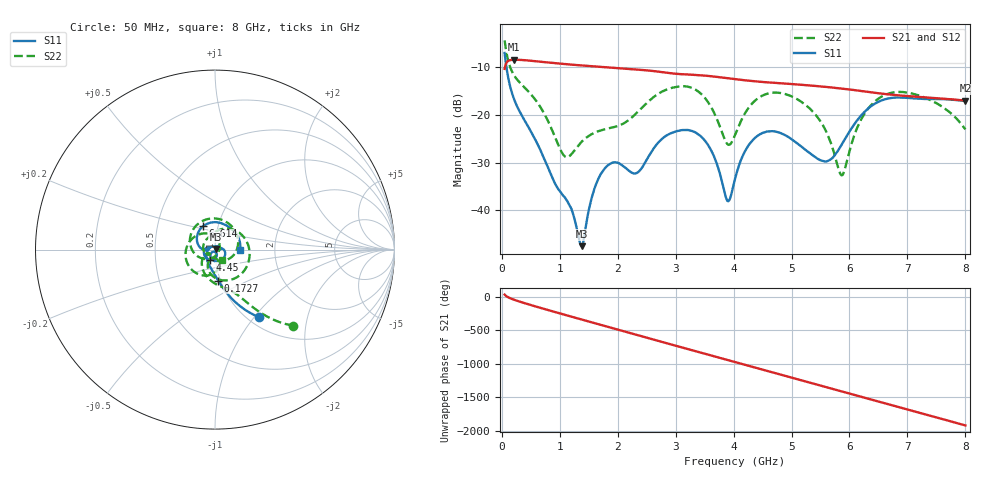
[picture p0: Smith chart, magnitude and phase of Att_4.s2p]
#  HZ  S  DB  R  50.00
! Rohde & Schwarz Vector Network Analyzer
! Rohde-Schwarz,ZNB40-4Port,1311601084101679,3.45
! Created: UTC 4/25/2025, 9:29:52 AM
! freq[Hz]  db:S11  ang:S11  db:S21  ang:S21  db:S12  ang:S12  db:S22  ang:S22
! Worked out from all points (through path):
!   1750 points, 50 MHz to 8 GHz, reference 50 ohm
!   highest |S21| = -8.37 dB at 213.6 MHz (marker M1); lowest = -17.0 dB at 8 GHz (marker M2)
!   group delay of S21, straight-line fit = 666 ps
!   lowest |S11| = -47.6 dB at 1.377 GHz (marker M3), VSWR 1.01, Z = 50.3 + j0.294 ohm
!   |S11| at or under -10 dB: 82.13 MHz to end of sweep
!   |S22| runs from -32.7 to -4.3 dB; largest |S21 - S12| = 0.00051
!   S11 on the Smith chart (normalised r, x): 50 MHz: 1.12, -1.06; 172.7 MHz: 0.98, -0.35; 4.45 GHz: 0.94, -0.11; 6.614 GHz: 0.85, +0.23; 8 GHz: 1.33, -0.01
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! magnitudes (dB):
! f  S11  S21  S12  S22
! 50 MHz  -7.0  -10.3  -10.3  -4.3
! 172.7 MHz  -15.2  -8.4  -8.4  -10.7
! 213.6 MHz  -16.7  -8.4  -8.4  -11.7
! 1.077 GHz  -37.2  -9.3  -9.3  -28.6
! 1.377 GHz  -47.6  -9.6  -9.6  -25.6
! 1.577 GHz  -36.3  -9.8  -9.8  -23.9
! 1.759 GHz  -31.5  -9.9  -9.9  -23.1
! 2.332 GHz  -32.2  -10.4  -10.4  -19.5
! 2.7 GHz  -25.8  -10.9  -10.9  -15.5
! 3.323 GHz  -23.5  -11.6  -11.6  -14.5
! 3.632 GHz  -27.9  -11.9  -11.9  -18.8
! 3.891 GHz  -38.0  -12.3  -12.3  -26.1
! 4.027 GHz  -33.3  -12.5  -12.5  -24.1
! 4.45 GHz  -24.1  -13.0  -13.0  -16.3
! 5.35 GHz  -28.3  -13.8  -13.8  -19.1
! 5.618 GHz  -29.7  -14.1  -14.1  -24.0
! 5.868 GHz  -26.2  -14.4  -14.4  -32.7
! 6.209 GHz  -20.0  -15.0  -15.0  -20.8
! 6.614 GHz  -16.7  -15.6  -15.6  -15.8
! 6.677 GHz  -16.5  -15.7  -15.7  -15.5
! 7.364 GHz  -16.6  -16.3  -16.3  -16.7
! 8 GHz  -17.1  -17.0  -17.0  -23.0
